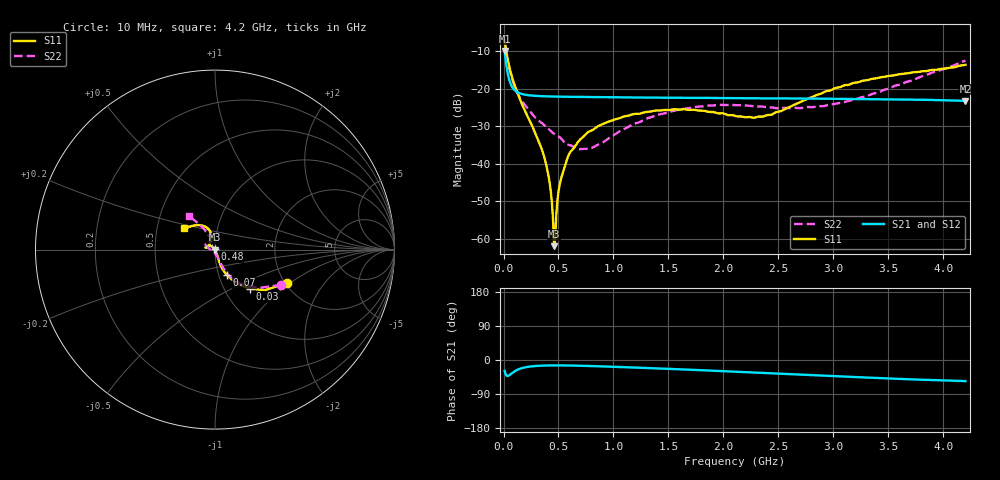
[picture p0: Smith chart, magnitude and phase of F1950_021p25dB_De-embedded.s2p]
! Integrated Device Technology
! Corporate Headquarters
! 6024 Silver Creek Valley Road
! San Jose, CA 95138  USA
! Phone:  1-408-284-8200
! Toll Free:  1-800-223-1366
! Webpage:  http://www.idt.com/
! Timing and RF Division
! 515 Groton Road, Suite 102
! Westford, MA 01886-6024
! Device:  F1950
! Description: 7-bit 0.25 dB Digital Step Attenuator
! Frequency:  150.0 -  4000.00 MHz
! Package:  4x4 mm Thin QFN Plastic Package: 24 pin
! Ports:  2 RF, 12 DC
!  Pin  1  = D0
!  Pin  2  = VDD
!  Pin  3  = Vmode
!  Pin  4  = GND
!  Pin  5  = RF1  =  Port 1
!  Pin  6  = GND
!  Pin  7  = GND
!  Pin  8  = GND
!  Pin  9  = GND
!  Pin 10  = GND
!  Pin 11  = GND
!  Pin 12  = GND
!  Pin 13  = GND
!  Pin 14  = RF2  =  Port 2
!  Pin 15  = GND
!  Pin 16  = LE
!  Pin 17  = CLK
!  Pin 18  = DATE
!  Pin 19  = D6
!  Pin 20  = D5
!  Pin 21  = D4
!  Pin 22  = D3
!  Pin 23  = D2
!  Pin 24  = D1
! State:  85
! Atten State:  21.25 dB
! Voltage:  +5.00 Volts
! Current:  Not Measured mA
! Data:  The device was measured on a the F195X evaluation board which has
!  individual transmission lines to the RF pins.  Data was collected
!  using a calibrated network analyzer.  The evaluation board was
!  de-embedded using a TRL calibration technique.
!  The reference plane is the edge of the package pin.
! Misc:  Board 2019
!  Action Tracker AT0250
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# GHz S dB R 50
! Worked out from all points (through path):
!   420 points, 10 MHz to 4.2 GHz, reference 50 ohm
!   highest |S21| = -9.88 dB at 10 MHz (marker M1); lowest = -23.2 dB at 4.2 GHz (marker M2)
!   group delay of S21, straight-line fit = 28.3 ps
!   lowest |S11| = -62.0 dB at 460 MHz (marker M3), VSWR 1.00, Z = 50 - j0.0717 ohm
!   |S11| at or under -10 dB: 26.13 MHz to end of sweep
!   |S22| runs from -36.1 to -7.6 dB; largest |S21 - S12| = 0.00013
!   S11 on the Smith chart (normalised r, x): 10 MHz: 2.05, -0.95; 30 MHz: 1.31, -0.63; 70 MHz: 1.09, -0.32; 480 MHz: 1.00, +0.00; 4.2 GHz: 0.69, +0.17
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0.01  -7.06 -24.8  -9.88 -28.5  -9.88 -28.5  -7.56 -27.9
0.03  -10.68 -48.3  -14.45 -41.8  -14.45 -41.8  -11.41 -48.8
0.07  -16.11 -64.8  -19.00 -36.2  -19.00 -36.1  -16.50 -63.1
0.16  -23.53 -71.0  -21.29 -22.1  -21.29 -22.1  -22.89 -70.0
0.37  -38.11 -65.0  -21.96 -14.7  -21.96 -14.7  -29.60 -76.0
0.42  -45.09 -70.3  -22.00 -14.3  -22.00 -14.3  -30.96 -77.7
0.45  -54.64 -82.7  -22.02 -14.3  -22.02 -14.2  -31.75 -81.4
0.46  -61.96 -116.0  -22.03 -14.2  -22.03 -14.2  -31.97 -82.7
0.48  -53.56 139.1  -22.04 -14.2  -22.04 -14.2  -32.31 -85.3
0.51  -45.62 133.7  -22.06 -14.2  -22.06 -14.3  -32.86 -87.3
0.56  -40.40 131.5  -22.08 -14.4  -22.08 -14.4  -34.38 -92.9
0.61  -36.74 133.8  -22.10 -14.6  -22.10 -14.6  -35.06 -103.5
0.71  -33.14 136.1  -22.14 -15.2  -22.14 -15.3  -36.02 -123.6
0.81  -30.96 139.6  -22.17 -16.1  -22.17 -16.1  -35.64 -146.9
0.99  -28.36 146.5  -22.23 -17.8  -22.23 -17.8  -32.55 -174.4
1.41  -25.76 162.7  -22.33 -22.4  -22.33 -22.4  -26.86 162.9
1.73  -25.56 168.2  -22.39 -26.1  -22.38 -26.1  -24.86 154.1
2.11  -27.24 157.6  -22.46 -31.0  -22.46 -31.0  -24.35 144.3
2.43  -26.91 125.3  -22.51 -34.9  -22.51 -34.9  -24.92 133.7
2.81  -22.14 104.6  -22.58 -39.9  -22.57 -39.9  -24.86 118.1
3.51  -16.50 117.0  -22.76 -48.8  -22.76 -48.8  -19.86 114.6
4.2  -13.54 145.6  -23.18 -55.7  -23.17 -55.7  -12.43 127.7
